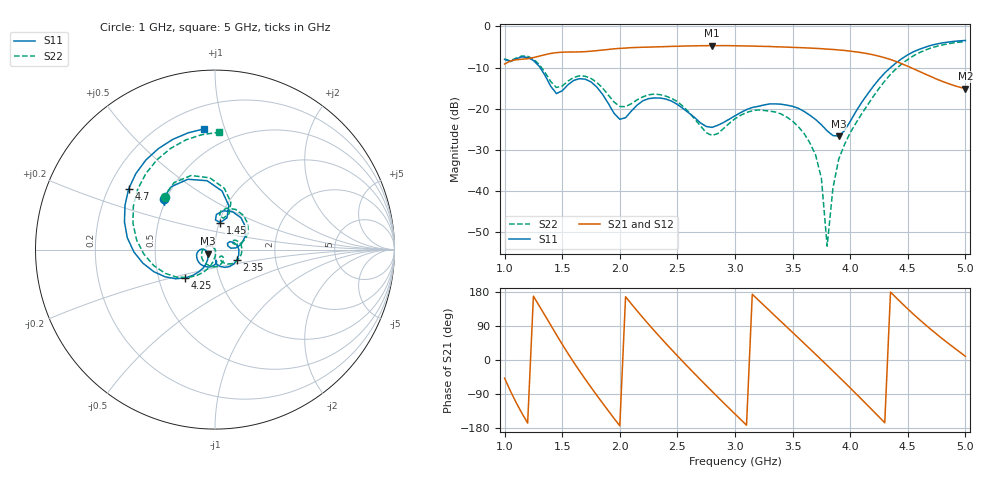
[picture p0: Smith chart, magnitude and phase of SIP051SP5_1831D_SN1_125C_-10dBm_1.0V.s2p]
# GHz  S  dB  R  50
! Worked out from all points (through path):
!   81 points, 1 GHz to 5 GHz, reference 50 ohm
!   highest |S21| = -4.66 dB at 2.8 GHz (marker M1); lowest = -15.1 dB at 5 GHz (marker M2)
!   lowest |S11| = -26.6 dB at 3.9 GHz (marker M3), VSWR 1.10, Z = 46.1 - j2.14 ohm
!   |S11| at or under -10 dB: 1.308 GHz to 4.349 GHz (3.042 GHz wide, 108 % of centre)
!   |S22| runs from -53.3 to -3.7 dB; largest |S21 - S12| = 0.0017
!   S11 on the Smith chart (normalised r, x): 1 GHz: 0.49, +0.33; 1.45 GHz: 1.01, +0.31; 2.35 GHz: 1.27, -0.15; 4.25 GHz: 0.69, -0.23; 4.7 GHz: 0.28, +0.29; 5 GHz: 0.35, +0.85
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1  -8.00 135.2  -9.13 -48.1  -9.12 -47.9  -7.88 133.1
1.1  -7.86 135.6  -8.09 -112.3  -8.10 -112.3  -7.69 131.9
1.25  -8.26 96.6  -7.56 168.4  -7.57 168.4  -7.94 94.2
1.45  -16.30 79.0  -6.36 66.6  -6.34 66.7  -14.83 74.9
1.7  -12.80 50.8  -6.12 -50.6  -6.11 -50.6  -12.10 50.5
1.85  -16.48 11.8  -5.74 -113.6  -5.73 -113.7  -14.93 19.0
2  -22.54 15.7  -5.33 -173.7  -5.32 -173.7  -19.44 18.5
2.2  -18.05 11.6  -5.06 111.9  -5.06 111.9  -17.10 17.2
2.35  -17.38 -25.7  -4.94 60.1  -4.93 60.3  -16.57 -10.0
2.55  -19.95 -70.4  -4.77 -4.9  -4.76 -5.0  -19.43 -48.7
2.8  -24.50 -84.4  -4.66 -82.7  -4.65 -82.7  -26.46 -50.9
3  -21.69 -89.3  -4.70 -142.6  -4.69 -142.6  -22.41 -52.2
3.2  -19.41 -117.7  -4.82 159.0  -4.82 159.0  -20.26 -95.5
3.4  -18.88 -148.8  -4.98 101.3  -4.97 101.3  -21.25 -148.6
3.7  -22.60 177.7  -5.33 15.0  -5.33 14.8  -31.21 133.9
3.75  -23.87 178.3  -5.40 0.3  -5.41 0.4  -36.84 125.1
3.8  -25.35 -177.6  -5.51 -14.2  -5.49 -14.2  -53.33 95.2
3.9  -26.62 -150.3  -5.72 -43.8  -5.71 -43.8  -32.25 -81.5
4.25  -12.83 -136.4  -7.24 -150.1  -7.21 -150.1  -15.05 -125.1
4.35  -9.99 -151.5  -8.04 179.2  -8.05 179.2  -11.63 -144.1
4.7  -4.61 144.8  -12.15 80.8  -12.17 80.8  -5.25 142.0
5  -3.41 95.0  -15.08 9.7  -15.10 9.7  -3.69 88.1
